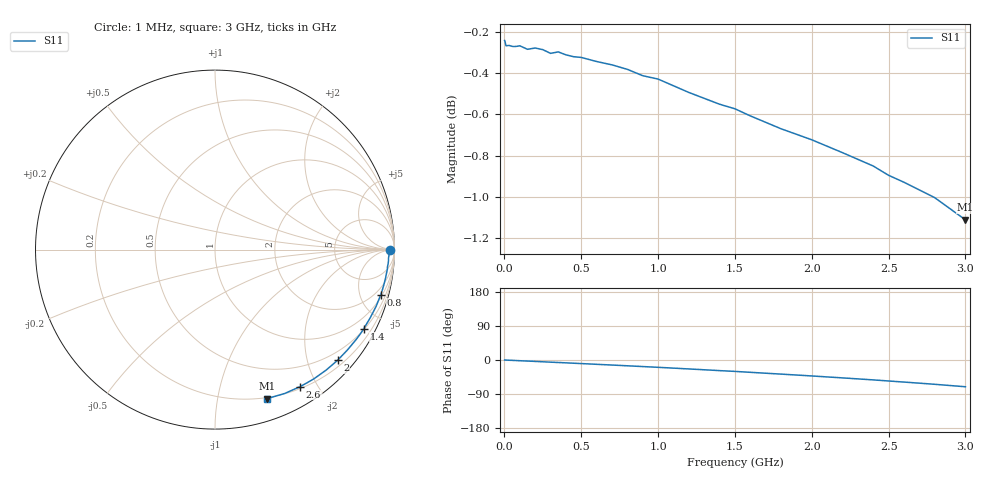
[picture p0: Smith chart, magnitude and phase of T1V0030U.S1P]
! SIEMENS Small Signal Semiconductors
! BAT68-04
! Si Schottky Diode (2 diodes in series, pin 3 open) in SOT23
! IF = 0.03 mA
! S-Parameters:  August  1994
# GHz  S  MA  R  50
!  f  S11
! GHz  MAG  ANG
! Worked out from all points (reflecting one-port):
!   33 points, 1 MHz to 3 GHz, reference 50 ohm
!   lowest |S11| = -1.1 dB at 3 GHz (marker M1), VSWR 15.64, Z = 9.5 - j69.8 ohm
!   phase of S11 starts at 0 deg and turns -71 deg over the sweep
!   S11 on the Smith chart (normalised r, x): 1 MHz: 72, +0; 800 MHz: 1.20, -7.25; 1.4 GHz: 0.53, -3.94; 2 GHz: 0.32, -2.56; 2.6 GHz: 0.22, -1.78; 3 GHz: 0.19, -1.40
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0.001  0.9727 0.0
0.003  0.9724 -0.1
0.01  0.9698 -0.2
0.03  0.97 -0.6
0.05  0.9695 -0.9
0.1  0.9698 -1.9
0.15  0.9679 -2.8
0.2  0.9686 -3.7
0.3  0.9657 -5.7
0.35  0.9665 -6.6
0.4  0.9649 -7.5
0.5  0.9635 -9.4
0.6  0.9613 -11.4
0.7  0.9595 -13.3
0.8  0.9571 -15.3
1  0.9519 -19.3
1.2  0.9448 -23.6
1.4  0.9386 -28.0
1.5  0.9362 -30.1
1.6  0.9325 -32.5
1.8  0.9258 -37.2
2  0.9201 -42.1
2.2  0.9135 -47.2
2.4  0.9067 -52.5
2.5  0.902 -55.4
2.6  0.8985 -58.2
2.8  0.8908 -64.1
3  0.8798 -70.6
